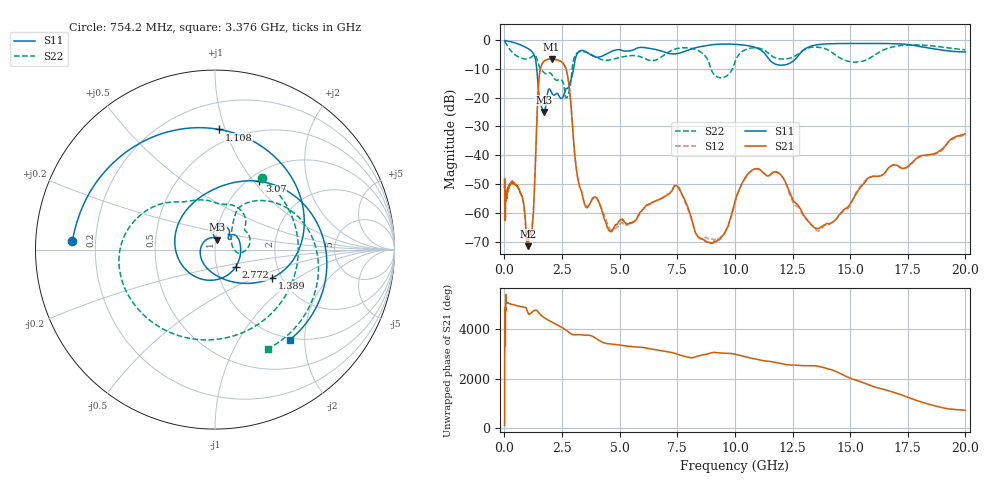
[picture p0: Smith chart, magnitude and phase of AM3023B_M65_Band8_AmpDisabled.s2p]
!Agilent Technologies,E8364B,MY43040894,A.07.50.67
!Agilent E8364B: A.07.50.67
!Date: Tuesday, October 27, 2020 10:50:11
!Correction: S11(Full 2 Port(1,2))
!S21(Full 2 Port(1,2))
!S12(Full 2 Port(1,2))
!S22(Full 2 Port(1,2))
!S2P File: Measurements: S11, S21, S12, S22:Log Frequency Sweep
# Hz S  dB  R 50
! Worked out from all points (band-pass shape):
!   3201 points, 10 MHz to 20 GHz, reference 50 ohm
!   highest |S21| = -6.67 dB at 2.05 GHz (marker M1); lowest = -71.5 dB at 1.02 GHz (marker M2)
!   |S21| within 3 dB of the highest: 1.574 GHz to 2.656 GHz (1.082 GHz wide, 51.2 % of centre)
!   lowest |S11| = -25.0 dB at 1.707 GHz (marker M3), VSWR 1.12, Z = 51 + j5.58 ohm
!   |S11| at or under -10 dB: 1.402 GHz to 3.002 GHz (1.6 GHz wide, 72.7 % of centre)
!   |S22| runs from -20.2 to -0.6 dB; largest |S21 - S12| = 0.0075
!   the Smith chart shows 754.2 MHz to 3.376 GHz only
!   S11 on the Smith chart (normalised r, x): 754.2 MHz: 0.11, +0.03; 1.108 GHz: 0.39, +0.95; 1.389 GHz: 1.79, -0.64; 2.772 GHz: 1.23, -0.24; 3.07 GHz: 1.12, +1.07; 3.376 GHz: 0.97, -1.69
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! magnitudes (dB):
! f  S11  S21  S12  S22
! 10 MHz  -0.3  -51.1  -57.5  -0.7
! 11.37 MHz  -0.3  -49.0  -48.8  -0.6
! 35.55 MHz  -0.4  -61.2  -61.3  -0.8
! 126.1 MHz  -0.5  -53.6  -52.9  -2.0
! 447.2 MHz  -1.1  -50.0  -49.7  -5.2
! 754.2 MHz  -2.0  -54.0  -54.2  -6.4
! 1.02 GHz  -3.0  -71.5  -69.0  -6.6
! 1.108 GHz  -3.5  -67.1  -66.1  -6.3
! 1.239 GHz  -4.5  -62.4  -61.0  -5.5
! 1.389 GHz  -9.0  -33.0  -33.0  -6.1
! 1.59 GHz  -22.7  -9.2  -9.2  -10.4
! 1.707 GHz  -25.0  -7.5  -7.6  -11.2
! 2.05 GHz  -18.3  -6.7  -6.7  -12.0
! 2.772 GHz  -16.5  -13.8  -13.9  -19.0
! 3.07 GHz  -6.9  -41.0  -41.2  -5.5
! 3.376 GHz  -3.7  -53.6  -53.6  -4.1
! 5.639 GHz  -3.4  -62.9  -62.9  -5.5
! 7.463 GHz  -4.9  -50.5  -50.2  -3.1
! 9.111 GHz  -1.7  -69.8  -69.1  -12.2
! 10.97 GHz  -2.9  -44.6  -44.8  -2.8
! 13.84 GHz  -1.5  -64.3  -64.6  -2.9
! 20 GHz  -4.2  -32.6  -33.0  -3.5
